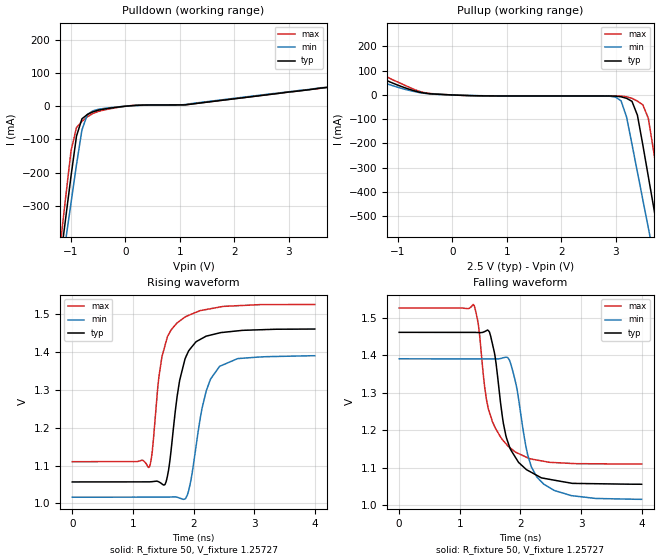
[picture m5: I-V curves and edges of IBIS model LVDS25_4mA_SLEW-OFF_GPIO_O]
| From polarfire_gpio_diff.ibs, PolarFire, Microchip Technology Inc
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|   Model LVDS25_4mA_SLEW-OFF_GPIO_O
[Model]   LVDS25_4mA_SLEW-OFF_GPIO_O
Model_type   Output
Polarity   Non-Inverting
Enable   Active-High
Vmeas =   1.2
Cref =   5p
Rref =   100
|   typ   min   max
C_comp_pullup   2.605e-12   2.605e-12   2.76e-12
C_comp_pulldown  2.605e-12   2.605e-12   2.76e-12
[Temperature Range]  25C   100C   -40C
[Voltage Range]  2.5   2.375   2.625
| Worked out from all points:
|   slope of the pulldown table from 0 to 0.375 V, typ, clamps not added: 106 ohm
|   slope of the pullup table from 0 to 0.375 V, typ, clamps not added: 130 ohm
|   rising waveform, R_fixture 50, V_fixture 1.25727: 20-80 % time 229ps typ, 263ps min, 225ps max; typ from 1.06 V to 1.46 V
|   falling waveform, R_fixture 50, V_fixture 1.25727: 20-80 % time 285ps typ, 282ps min, 298ps max; typ from 1.46 V to 1.06 V
[Pulldown]
|Voltage   I(typ)   I(min)   I(max)
-2.5V     -2.163A    -2.027A    -2.344A
-1.2V     -468.8mA   -521.4mA   -422.9mA
-1.1V     -339.5mA   -406.4mA   -276.5mA
-1V       -210.3mA   -291.3mA   -134.2mA
-900mV    -90.3mA    -176.4mA   -64.32mA
-800mV    -38.14mA   -71.66mA   -45.84mA
-700mV    -24.92mA   -24.97mA   -32.1mA
-600mV    -17.06mA   -14.08mA   -22.08mA
100mV     1.398mA    1.072mA    1.786mA
3.7V      56.63mA    56.44mA    56.88mA
3.9V      60.06mA    66.45mA    73.01mA
5V        214mA      191.7mA    236.8mA
[Pullup]
|Voltage   I(typ)   I(min)   I(max)
-2.5V     229.4mA    189.2mA    276mA
-1.5V     90.6mA     72.23mA    112.6mA
-500mV    7.398mA    6.365mA    8.936mA
2.9V      -4.261mA   -5.325mA   -4.256mA
3.1V      -7.624mA   -24.26mA   -4.733mA
3.2V      -13.72mA   -90.63mA   -7.241mA
3.4V      -83.58mA   -318mA     -25.16mA
3.6V      -335.9mA   -547.8mA   -95.77mA
3.8V      -594.4mA   -777.6mA   -381mA
3.9V      -723.8mA   -892.5mA   -527.3mA
4V        -853.2mA   -1.008A    -673.7mA
5V        -2.158A    -2.169A    -2.15A
[Ramp]
| variable   typ   min   max
dV/dt_r 0.2476/0.2305e-9   0.2281/0.2644e-9   0.2588/0.2227e-9
dV/dt_f 0.2468/0.2839e-9   0.2272/0.2834e-9   0.2553/0.2952e-9
R_load = 50
[Rising waveform]
R_fixture= 50
V_fixture= 1.25727
V_fixture_min= 1.19545
V_fixture_max= 1.31876
|Time   V(typ)   V(min)   V(max)
0s        1.057V     1.017V     1.111V
1.27ns    1.057V     1.017V     1.096V
1.32ns    1.058V     1.017V     1.138V
1.43ns    1.057V     1.017V     1.336V
1.53ns    1.05V      1.017V     1.418V
1.77ns    1.325V     1.014V     1.483V
1.87ns    1.387V     1.013V     1.494V
2.2ns     1.442V     1.293V     1.513V
2.43ns    1.451V     1.363V     1.52V
4ns       1.462V     1.391V     1.526V
[Falling waveform]
R_fixture= 50
V_fixture= 1.25727
V_fixture_min= 1.19545
V_fixture_max= 1.31876
|Time   V(typ)   V(min)   V(max)
0s        1.462V     1.391V     1.526V
1.23ns    1.462V     1.391V     1.535V
1.31ns    1.461V     1.391V     1.478V
1.47ns    1.466V     1.391V     1.259V
1.58ns    1.4V       1.391V     1.209V
1.76ns    1.187V     1.395V     1.165V
1.91ns    1.13V      1.336V     1.143V
2.12ns    1.094V     1.135V     1.127V
2.38ns    1.073V     1.058V     1.118V
4ns       1.056V     1.016V     1.111V
